//{attribute 'qualified_only'}
{attribute 'strict'}
TYPE E_STLAutomaticActiveState :
(
	eSTLAutoActive_Red 			:= 0,
	eSTLAutoActive_YellowRed	:= 1,
	eSTLAutoActive_Green 		:= 2,
	eSTLAutoActive_Yellow		:= 3 
);
END_TYPE
